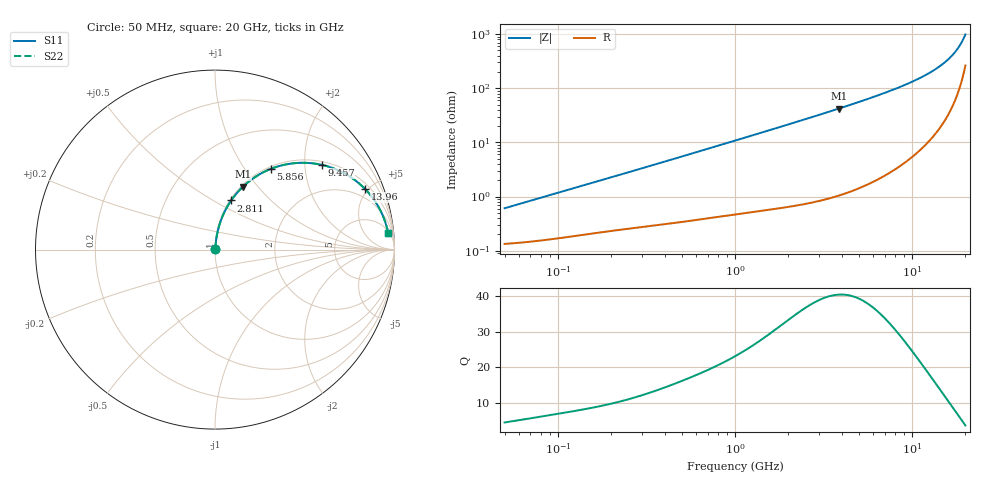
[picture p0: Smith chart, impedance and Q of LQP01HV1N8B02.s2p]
!Murata Part Number: LQP01HV1N8B02
!These Parameters are Measured in Series Mode Connection
!  o--[Z]--o
!Port1  Port2
!  o-------o
!Freq. Start=50[MHz] Stop=20[GHz], 401[Steps]
# Hz S RI R 50
!Freq.(Hz) S11(Real) S11(Imag) S21(Real) S21(Imag) S12(Real) S12(Imag) S22(Real) S22(Imag)
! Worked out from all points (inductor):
!   401 points, 50 MHz to 20 GHz, reference 50 ohm
!   read as one part in series: L = 1.88 nH near 51.52 MHz
!   highest Q = 40.5 at 3.85 GHz (marker M1), where L = 1.74 nH
!   S11 on the Smith chart (normalised r, x): 50 MHz: 1.00, +0.01; 2.811 GHz: 1.02, +0.61; 5.856 GHz: 1.04, +1.33; 9.457 GHz: 1.09, +2.43; 13.96 GHz: 1.33, +4.80; 20 GHz: 6, +19
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5e7  0.00136 0.00591  0.9986 -0.00591  0.9986 -0.00591  0.00136 0.00591
1.364002e8  0.00218 0.0156  0.9978 -0.0156  0.9978 -0.0156  0.00218 0.0156
3.721004e8  0.00464 0.0407  0.9954 -0.0407  0.9954 -0.0407  0.00464 0.0407
6.285508e8  0.00834 0.0675  0.9917 -0.0675  0.9917 -0.0675  0.00834 0.0675
1e9  0.016 0.1056  0.984 -0.1056  0.984 -0.1056  0.016 0.1056
1.689197e9  0.0371 0.1734  0.9629 -0.1734  0.9629 -0.1734  0.0371 0.1734
2.728004e9  0.0856 0.2668  0.9144 -0.2668  0.9144 -0.2668  0.0856 0.2668
2.810964e9  0.0902 0.2737  0.9098 -0.2737  0.9098 -0.2737  0.0902 0.2737
3.850025e9  0.1564 0.3511  0.8436 -0.3511  0.8436 -0.3511  0.1564 0.3511
4.748272e9  0.223 0.4039  0.777 -0.4039  0.777 -0.4039  0.223 0.4039
5.856089e9  0.3117 0.45  0.6883 -0.45  0.6883 -0.45  0.3117 0.45
7.442007e9  0.4412 0.4814  0.5588 -0.4814  0.5588 -0.4814  0.4412 0.4814
8.389408e9  0.5154 0.4831  0.4846 -0.4831  0.4846 -0.4831  0.5154 0.4831
9.457416e9  0.5935 0.4725  0.4065 -0.4725  0.4065 -0.4725  0.5935 0.4725
1.166392e10  0.7306 0.4194  0.2694 -0.4194  0.2694 -0.4194  0.7306 0.4194
1.276073e10  0.7857 0.3826  0.2143 -0.3826  0.2143 -0.3826  0.7857 0.3826
1.396067e10  0.8363 0.3374  0.1637 -0.3374  0.1637 -0.3374  0.8363 0.3374
1.573793e10  0.8941 0.2656  0.1059 -0.2656  0.1059 -0.2656  0.8941 0.2656
1.721783e10  0.9283 0.2042  0.0717 -0.2042  0.0717 -0.2042  0.9283 0.2042
1.828096e10  0.9462 0.1605  0.0538 -0.1605  0.0538 -0.1605  0.9462 0.1605
1.940974e10  0.9598 0.115  0.0402 -0.115  0.0402 -0.115  0.9598 0.115
2e10  0.965 0.0917  0.035 -0.0917  0.035 -0.0917  0.965 0.0917
